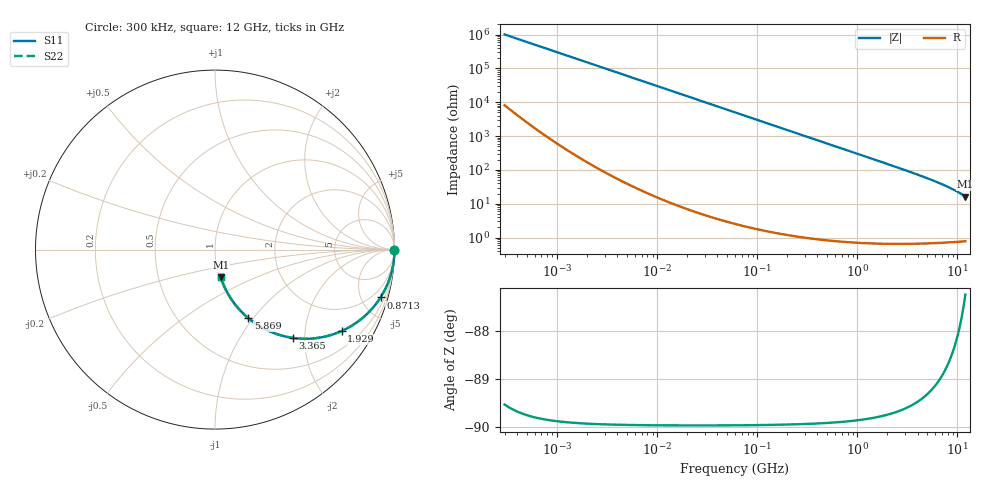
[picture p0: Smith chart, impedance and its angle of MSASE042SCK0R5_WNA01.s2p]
! MSASE042SCK0R5_WNA01  S-PARAMETER MODEL  ( General Type )
! Model Generated by TAIYO YUDEN Corporation (http://www.ty-top.com)
! Version 2.0
! TAIYO YUDEN Control No. 120810
! Copyright(c) 2011 TAIYO YUDEN CO.,LTD. All Rights Reserved.
! Product Description (link to TY-COMPAS)
! https://ds.yuden.co.jp/TYCOMPAS/or/detail?pn=MSASE042SCK0R5AWNA01&u=M
! Products Name : Multilayer Ceramic Capacitors
! Characteristics :
!  Capacitance : 0.5 pF , Rated Voltage : 16V , TCC : CK / C0K
!  Case Size : 0.4 x 0.2 / 0.016 x 0.008 [mm/inch] , Thickness : 0.2 / 0.008 [mm/inch]
!  (Conditions: Temperature = 25 degC , DC Bias Current/Voltage = 0A / 0V)
! External Node Assignments :
!  1  o---| |---o  2
! GND o---------o GND
! Frequency Range : 0.3MHz  -  12000MHz  [ 401 STEP ]
# MHz S RI R 50
! Freq[MHz].  S11 Real  S11 Imag  S21 Real  S21 Imag  S12 Real  S12 Imag  S22 Real  S22 Imag
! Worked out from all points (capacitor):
!   401 points, 300 kHz to 12 GHz, reference 50 ohm
!   read as one part in series: C = 527 fF near 316.3 kHz
!   lowest |Z| = 16.2 ohm at 12 GHz (marker M1)
!   S11 on the Smith chart (normalised r, x): 300 kHz: open; 871.3 MHz: 1.01, -6.92; 1.929 GHz: 1.01, -3.10; 3.365 GHz: 1.01, -1.75; 5.869 GHz: 1.01, -0.94; 12 GHz: 1.02, -0.32
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0.3  1 -9.93e-05  8.13e-07 9.93e-05  8.13e-07 9.93e-05  1 -9.93e-05
0.324815  1 -0.000107  7.92e-07 0.000107  7.92e-07 0.000107  1 -0.000107
1.769972  1 -0.000586  1.06e-06 0.000586  1.06e-06 0.000586  1 -0.000586
10.44266  1 -0.00346  1.37e-05 0.00346  1.37e-05 0.00346  1 -0.00346
60  0.9996 -0.0198  0.000404 0.0198  0.000404 0.0198  0.9996 -0.0198
164.1901  0.997 -0.0542  0.00298 0.0542  0.00298 0.0542  0.997 -0.0542
353.9943  0.9863 -0.1156  0.0137 0.1156  0.0137 0.1156  0.9863 -0.1156
555.3718  0.967 -0.1778  0.033 0.1778  0.033 0.1778  0.967 -0.1778
871.3074  0.9225 -0.2663  0.0775 0.2663  0.0775 0.2663  0.9225 -0.2663
1076.992  0.8861 -0.3164  0.1139 0.3164  0.1139 0.3164  0.8861 -0.3164
1331.232  0.8356 -0.3692  0.1644 0.3692  0.1644 0.3692  0.8356 -0.3692
1602.47  0.7775 -0.4141  0.2225 0.4141  0.2225 0.4141  0.7775 -0.4141
1928.972  0.7059 -0.4535  0.2941 0.4535  0.2941 0.4535  0.7059 -0.4535
2088.533  0.6713 -0.4675  0.3287 0.4675  0.3287 0.4675  0.6713 -0.4675
2650.866  0.5562 -0.4939  0.4438 0.4939  0.4438 0.4939  0.5562 -0.4939
3364.605  0.433 -0.4918  0.567 0.4918  0.567 0.4918  0.433 -0.4918
4385.161  0.3028 -0.4544  0.6972 0.4544  0.6972 0.4544  0.3028 -0.4544
5868.704  0.185 -0.3811  0.815 0.3811  0.815 0.3811  0.185 -0.3811
7064.448  0.1277 -0.3245  0.8723 0.3245  0.8723 0.3245  0.1277 -0.3245
8503.825  0.0839 -0.265  0.9161 0.265  0.9161 0.265  0.0839 -0.265
9708.23  0.0599 -0.2223  0.9401 0.2223  0.9401 0.2223  0.0599 -0.2223
12000  0.0326 -0.155  0.9674 0.155  0.9674 0.155  0.0326 -0.155
